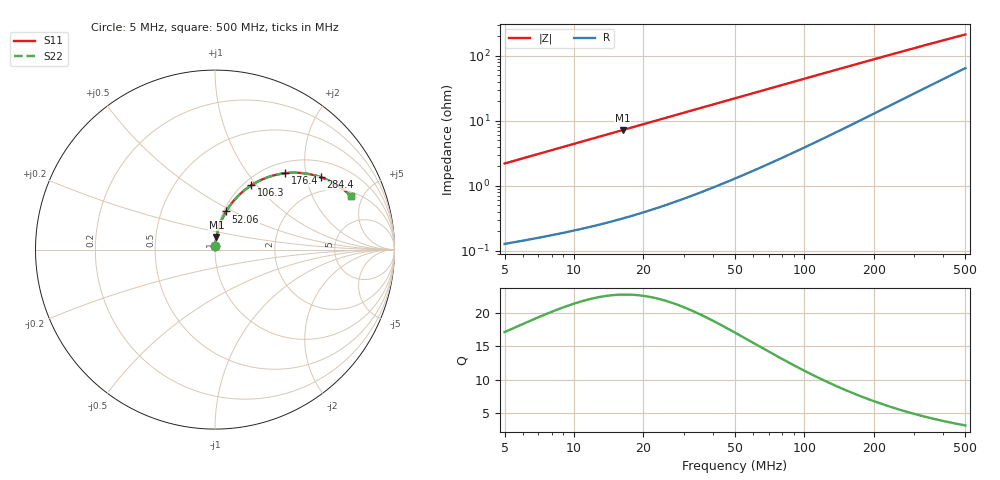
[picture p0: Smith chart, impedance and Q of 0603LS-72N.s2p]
# MHz S MA R 50
!Freq  MagS11  AngS11  MagS21  AngS21  MagS12  AngS12  MagS22  AngS22
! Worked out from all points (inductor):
!   801 points, 5 MHz to 500 MHz, reference 50 ohm
!   read as one part in series: L = 70 nH near 5.116 MHz
!   highest Q = 22.8 at 16.27 MHz (marker M1), where L = 70.2 nH
!   S11 on the Smith chart (normalised r, x): 5 MHz: 1.00, +0.04; 52.06 MHz: 1.03, +0.46; 106.3 MHz: 1.09, +0.93; 176.4 MHz: 1.21, +1.54; 284.4 MHz: 1.48, +2.43; 500 MHz: 2.28, +4.02
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5  0.022 85.4  0.9985 -1.3  0.9985 -1.3  0.022 85.4
7.14447  0.03142 85.3  0.9979 -1.8  0.9979 -1.8  0.03142 85.3
9.637625  0.04237 84.9  0.9971 -2.4  0.9971 -2.4  0.04237 84.9
12.70486  0.05583 84.2  0.996 -3.2  0.996 -3.2  0.05583 84.2
16.27309  0.07145 83.4  0.9943 -4.1  0.9943 -4.1  0.07145 83.4
19.3406  0.08482 82.6  0.9927 -4.9  0.9927 -4.9  0.08482 82.6
22.85441  0.1001 81.7  0.9905 -5.7  0.9905 -5.7  0.1001 81.7
30.82975  0.1342 79.5  0.9845 -7.7  0.9845 -7.7  0.1342 79.5
40.64153  0.1753 76.9  0.9752 -10.1  0.9752 -10.1  0.1753 76.9
52.05591  0.2215 73.8  0.962 -12.8  0.962 -12.8  0.2215 73.8
68.62305  0.2849 69.5  0.939 -16.5  0.939 -16.5  0.2849 69.5
87.89618  0.3526 64.8  0.9078 -20.6  0.9078 -20.6  0.3526 64.8
106.2845  0.4106 60.6  0.875 -24.1  0.875 -24.1  0.4106 60.6
135.3537  0.4895 54.7  0.8205 -29.1  0.8205 -29.1  0.4895 54.7
170.4002  0.5656 48.5  0.755 -34.1  0.755 -34.1  0.5656 48.5
176.3884  0.5768 47.5  0.7441 -34.9  0.7441 -34.9  0.5768 47.5
214.5211  0.6376 42.1  0.6785 -39.0  0.6785 -39.0  0.6376 42.1
253.4954  0.6845 37.5  0.6186 -42.4  0.6186 -42.4  0.6845 37.5
284.4265  0.7134 34.5  0.5766 -44.4  0.5766 -44.4  0.7134 34.5
336.1012  0.7502 30.2  0.5162 -47.0  0.5162 -47.0  0.7502 30.2
418.2828  0.7889 25.2  0.441 -49.6  0.441 -49.6  0.7889 25.2
500  0.8132 21.5  0.3851 -50.8  0.3851 -50.8  0.8132 21.5
